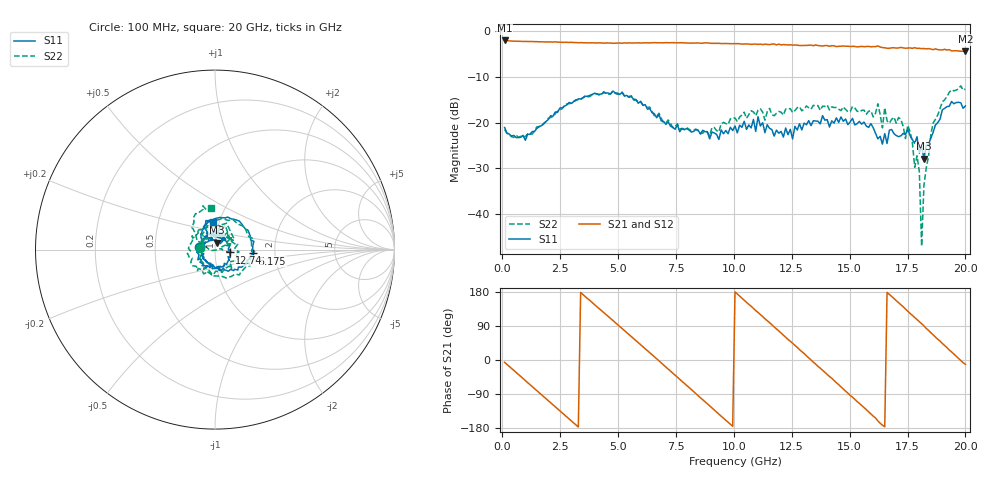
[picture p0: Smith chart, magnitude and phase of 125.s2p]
!Agilent Technologies,N5230C,MY49001569,A.09.33.09
!Agilent N5230C: A.09.33.09
!Date: Tuesday, July 28, 2015 18:48:41
!Correction: S11(Full 2 Port(1,2))
!S21(Full 2 Port(1,2))
!S12(Full 2 Port(1,2))
!S22(Full 2 Port(1,2))
!S2P File: Measurements: S11, S21, S12, S22:
# Hz S  dB  R 50
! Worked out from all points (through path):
!   201 points, 100 MHz to 20 GHz, reference 50 ohm
!   highest |S21| = -1.98 dB at 100 MHz (marker M1); lowest = -4.4 dB at 20 GHz (marker M2)
!   group delay of S21, straight-line fit = 151 ps
!   lowest |S11| = -27.9 dB at 18.21 GHz (marker M3), VSWR 1.08, Z = 50.8 + j3.96 ohm
!   |S11| at or under -10 dB: start of sweep to end of sweep
!   |S22| runs from -47.2 to -11.9 dB; largest |S21 - S12| = 0.02
!   S11 on the Smith chart (normalised r, x): 100 MHz: 0.84, +0.02; 5.175 GHz: 1.54, -0.07; 12.74 GHz: 1.18, -0.04; 20 GHz: 0.93, +0.29
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1e8  -21.10 170.8  -1.98 -6.2  -1.99 -5.9  -21.54 173.1
1.692e9  -20.70 142.4  -2.27 -91.6  -2.30 -91.7  -20.73 138.3
2.687e9  -16.38 107.7  -2.38 -144.9  -2.39 -144.8  -16.31 100.2
3.483e9  -14.59 71.6  -2.48 172.7  -2.48 172.7  -14.54 62.0
5.1745e9  -13.39 -5.8  -2.60 83.3  -2.59 83.4  -13.33 -24.7
6.7665e9  -18.29 -73.9  -2.50 -2.2  -2.49 -2.3  -17.96 -120.2
8.458e9  -21.68 -140.8  -2.52 -94.0  -2.59 -94.1  -21.84 130.0
1.005e10  -20.74 136.7  -2.66 179.7  -2.71 179.8  -19.01 32.2
1.15425e10  -21.28 54.2  -2.90 98.5  -2.76 98.8  -16.90 -49.8
1.27365e10  -21.64 -11.2  -3.01 33.3  -3.03 32.3  -16.75 -113.4
1.3433e10  -19.61 -61.2  -3.13 -5.6  -3.08 -5.6  -16.23 -144.4
1.49255e10  -20.48 -143.8  -3.25 -87.4  -3.19 -86.9  -17.64 144.8
1.6219e10  -23.59 141.7  -3.16 -160.6  -3.22 -160.2  -15.89 66.4
1.67165e10  -21.68 105.9  -3.71 173.2  -3.59 173.7  -20.14 43.9
1.75125e10  -21.50 55.3  -3.64 128.7  -3.72 128.6  -20.63 20.1
1.7811e10  -24.56 46.4  -3.56 112.1  -3.74 112.3  -29.85 19.6
1.79105e10  -23.13 56.1  -3.72 106.7  -3.67 106.8  -27.31 -2.0
1.801e10  -26.73 47.3  -3.71 101.2  -3.70 100.9  -30.72 9.5
1.81095e10  -25.15 62.1  -3.77 95.8  -3.65 95.0  -47.16 -44.8
1.8209e10  -27.94 75.9  -3.75 90.2  -3.85 89.0  -33.84 -165.6
1.8607e10  -22.15 127.9  -4.01 66.2  -3.85 66.3  -20.12 153.6
2e10  -16.36 94.1  -4.38 -11.5  -4.39 -12.0  -12.67 95.6
